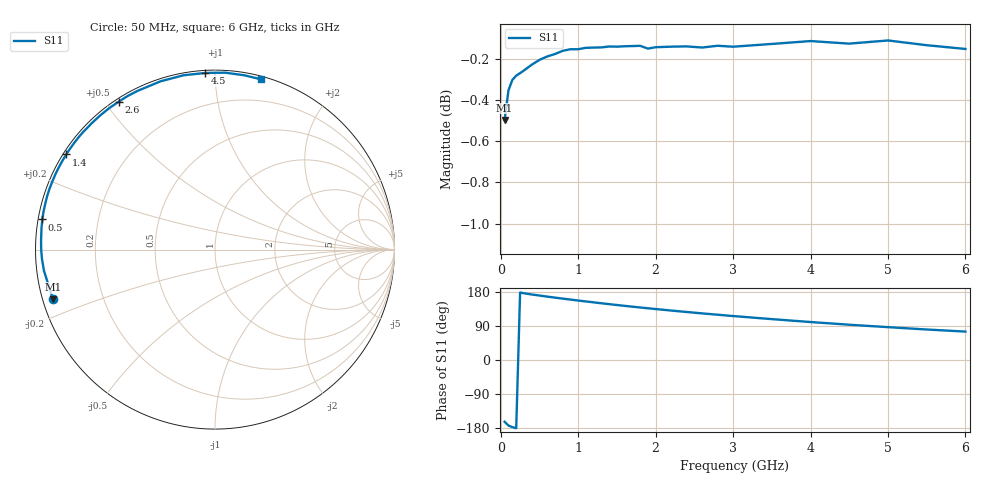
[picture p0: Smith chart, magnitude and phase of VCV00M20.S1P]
! Infineon Technologies  Discrete & RF Semiconductors
! BBY 56-03
! Si Tuning Diode in SOD323
! VR =
! S-Parameters:  June  1999
# GHz  S  MA  R  50
!  f  S11
! GHz  MAG  ANG
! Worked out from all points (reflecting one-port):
!   34 points, 50 MHz to 6 GHz, reference 50 ohm
!   lowest |S11| = -0.5 dB at 50 MHz (marker M1), VSWR 34.95, Z = 1.46 - j7.51 ohm
!   phase of S11 starts at -163 deg and turns -122 deg over the sweep
!   S11 on the Smith chart (normalised r, x): 50 MHz: 0.03, -0.15; 500 MHz: 0.01, +0.09; 1.4 GHz: 0.01, +0.29; 2.6 GHz: 0.01, +0.54; 4.5 GHz: 0.01, +0.95; 6 GHz: 0.02, +1.30
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0.05  0.9444 -162.9
0.1  0.9603 -173.0
0.15  0.9658 -177.2
0.2  0.9681 -179.9
0.25  0.9695 178.0
0.3  0.971 176.1
0.4  0.9741 172.9
0.5  0.9767 170.1
0.6  0.9786 167.3
0.8  0.9817 162.0
1  0.9826 156.9
1.1  0.9833 154.5
1.3  0.9836 149.7
1.4  0.9841 147.4
1.6  0.9842 142.9
1.8  0.9845 138.6
2  0.9837 134.5
2.2  0.984 130.5
2.4  0.9841 126.7
2.6  0.9835 123.0
2.8  0.9845 119.5
3  0.9839 116.0
3.5  0.9855 107.9
4  0.9871 100.2
4.5  0.9857 93.1
5  0.9874 86.7
5.5  0.9848 80.5
6  0.9827 75.0
